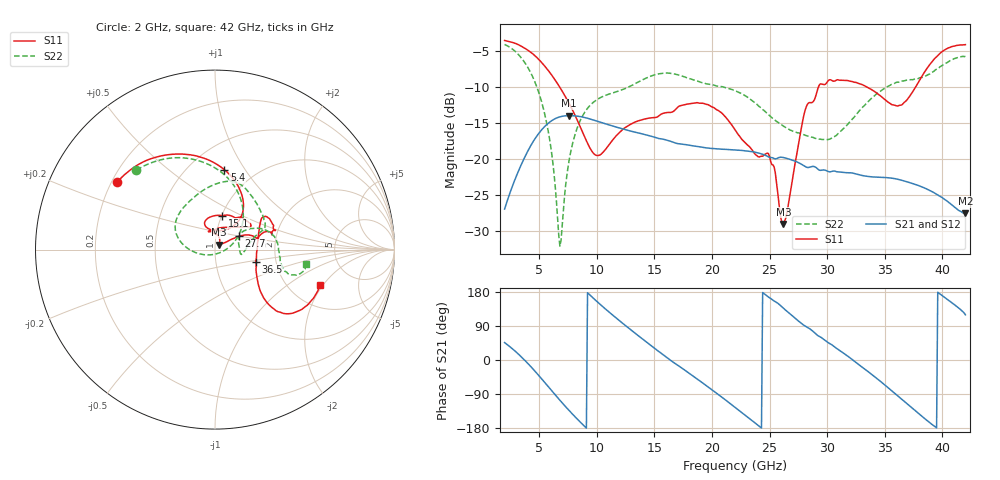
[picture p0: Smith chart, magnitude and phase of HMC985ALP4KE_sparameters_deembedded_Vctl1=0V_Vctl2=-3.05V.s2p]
!s2p File: Measurements: S11, S21, S12, S22
# GHz S dB R 50.0
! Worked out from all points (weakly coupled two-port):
!   401 points, 2 GHz to 42 GHz, reference 50 ohm
!   highest |S21| = -14.02 dB at 7.6 GHz (marker M1); lowest = -27.6 dB at 42 GHz (marker M2)
!   lowest |S11| = -29.1 dB at 26.2 GHz (marker M3), VSWR 1.07, Z = 52.3 + j2.8 ohm
!   |S11| at or under -10 dB: 6.761 GHz to 29.26 GHz (22.49 GHz wide, 125 % of centre); 33.39 GHz to 37.7 GHz (4.301 GHz wide, 12.1 % of centre)
!   |S22| runs from -32.2 to -4.1 dB; largest |S21 - S12| = 0.00068
!   S11 on the Smith chart (normalised r, x): 2 GHz: 0.22, +0.30; 5.4 GHz: 0.73, +0.81; 15.1 GHz: 1.01, +0.39; 27.7 GHz: 1.29, +0.20; 36.5 GHz: 1.57, -0.22; 42 GHz: 2.92, -1.90
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2  -3.57 145.5  -27.01 46.0  -27.00 45.9  -4.12 134.6
3.5  -4.42 119.7  -20.64 6.8  -20.67 6.8  -6.10 98.6
5.4  -6.98 83.3  -15.67 -56.4  -15.69 -56.4  -13.25 44.7
6.1  -8.41 70.5  -14.71 -81.5  -14.71 -81.5  -19.44 19.0
6.8  -10.10 59.9  -14.19 -106.2  -14.18 -106.2  -32.17 -70.1
7.6  -12.33 52.0  -14.02 -133.3  -14.04 -133.3  -20.23 -167.4
8.7  -16.07 53.4  -14.19 -167.9  -14.18 -167.9  -14.26 167.8
10.1  -19.56 87.1  -14.83 152.1  -14.82 152.1  -11.71 148.7
15.1  -14.28 78.1  -17.07 28.7  -17.05 28.7  -8.32 81.6
15.4  -14.04 74.5  -17.21 22.1  -17.21 22.1  -8.21 78.6
19.2  -12.30 33.6  -18.43 -60.7  -18.43 -60.8  -9.45 42.7
22  -15.96 52.0  -18.78 -124.8  -18.81 -124.8  -10.56 23.1
25  -19.73 99.7  -19.83 164.3  -19.80 164.3  -14.03 11.4
26.2  -29.07 49.5  -19.85 136.7  -19.88 136.7  -15.48 -1.0
27.7  -16.28 28.9  -20.71 98.2  -20.72 98.1  -16.53 -10.3
28.7  -12.19 13.0  -21.09 77.4  -21.09 77.4  -17.02 -6.4
31  -9.06 23.2  -21.85 27.0  -21.85 27.0  -16.45 27.3
33.3  -9.91 34.2  -22.42 -24.9  -22.41 -24.9  -12.51 29.7
35.4  -12.26 11.8  -22.68 -76.0  -22.66 -76.0  -9.86 17.0
36.5  -12.50 -16.5  -23.02 -104.4  -23.04 -104.3  -9.21 8.8
39.5  -5.84 -43.5  -24.95 -179.0  -24.90 -179.1  -7.56 -17.4
42  -4.15 -18.8  -27.59 119.2  -27.59 119.2  -5.76 -8.8
